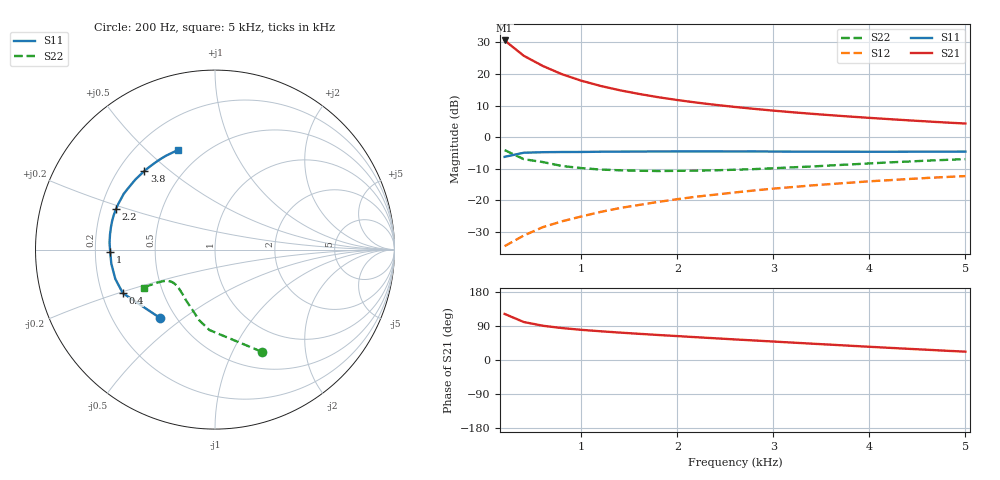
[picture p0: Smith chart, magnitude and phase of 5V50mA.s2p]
#  HZ  S  MA  R  50.0000
! Device:MCH4020
! Bias:VCE=5V, IC=50mA
!MHZ	S11(MAG/ANG)		S21(MAG/ANG)		S12(MAG/ANG)		S22(MAG/ANG)
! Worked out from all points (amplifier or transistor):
!   25 points, 200 Hz to 5 kHz, reference 50 ohm
!   highest |S21| = 30.5 dB at 200 Hz (marker M1)
!   |S21| within 3 dB of that: start of sweep to 323.8 Hz
!   unconditionally stable (mu >= 1): nowhere
!   at 1 kHz: K = 0.88, MSG = 21.4 dB, |S12| = -25.0 dB
!   at 2.6 kHz: K = 1.00, MSG = 13.5 dB, |S12| = -17.5 dB
!   at 5 kHz: K = 0.94, MSG = 8.3 dB, |S12| = -12.3 dB
!   S11 on the Smith chart (normalised r, x): 200 Hz: 0.41, -0.41; 400 Hz: 0.29, -0.21; 1 kHz: 0.26, -0.01; 2.2 kHz: 0.26, +0.18; 3.8 kHz: 0.31, +0.41; 5 kHz: 0.37, +0.63
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200  0.489 -128.9  33.66 121.6  0.019 61.0  0.625 -65.5
400  0.568 -154.7  19.27 100.2  0.028 61.3  0.449 -94.0
600  0.579 -163.6  13.27 90.3  0.038 64.6  0.404 -102.5
800  0.583 -172.3  9.829 84.2  0.047 66.7  0.35 -112.6
1000  0.584 -178.7  7.784 79.6  0.056 67.8  0.325 -119.9
1200  0.589 176.2  6.443 75.8  0.066 68.5  0.308 -125.6
1400  0.591 171.8  5.505 72.3  0.076 68.4  0.3 -129.7
1600  0.593 167.9  4.817 69.1  0.085 68.1  0.295 -133.2
1800  0.595 164.3  4.28 66.0  0.095 67.6  0.292 -136.3
2000  0.596 161.2  3.857 63.1  0.105 67.0  0.294 -138.9
2200  0.596 157.8  3.517 60.1  0.115 66.1  0.296 -141.1
2400  0.596 154.7  3.234 57.2  0.124 65.1  0.3 -142.9
2600  0.595 151.7  3 54.3  0.134 63.9  0.306 -144.7
2800  0.596 148.5  2.799 51.5  0.144 62.8  0.313 -145.9
3000  0.593 145.4  2.625 48.7  0.154 61.6  0.323 -147.3
3200  0.591 142.2  2.472 45.9  0.163 60.2  0.334 -148.3
3400  0.591 138.8  2.34 43.1  0.173 59.0  0.344 -149.0
3800  0.589 131.9  2.114 37.6  0.191 56.2  0.371 -150.2
4200  0.588 124.7  1.929 32.2  0.209 53.1  0.399 -150.9
4400  0.589 121.1  1.847 29.6  0.218 51.7  0.412 -151.3
4800  0.59 113.9  1.702 24.4  0.235 48.6  0.438 -151.7
5000  0.592 110.6  1.642 22.0  0.243 47.0  0.45 -152.0
